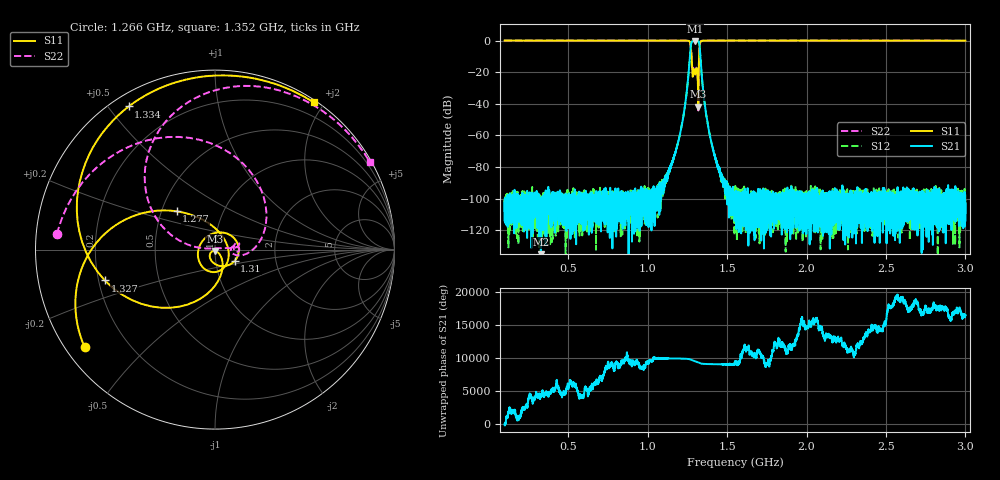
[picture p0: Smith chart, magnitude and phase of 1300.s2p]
# Hz S DB R 50
! Planar, S50180, 20087770, 20.1.2/1
! Date: 23.06.2021 14:42:37
! Data: Format (Calibration Info)
! Freq	S11:dB/Ang(F2)	S21:dB/Ang(F2)	S12:dB/Ang(F2)	S22:dB/Ang(F2)
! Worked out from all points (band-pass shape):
!   8991 points, 100 MHz to 3 GHz, reference 50 ohm
!   highest |S21| = -0.42 dB at 1.299 GHz (marker M1); lowest = -138.1 dB at 328.1 MHz (marker M2)
!   |S21| within 3 dB of the highest: 1.272 GHz to 1.327 GHz (55.52 MHz wide, 4.27 % of centre)
!   lowest |S11| = -41.8 dB at 1.319 GHz (marker M3), VSWR 1.02, Z = 49.9 - j0.794 ohm
!   |S11| at or under -10 dB: 1.277 GHz to 1.324 GHz (47.72 MHz wide, 3.67 % of centre)
!   |S22| runs from -44.2 to 0.0 dB; largest |S21 - S12| = 0.0016
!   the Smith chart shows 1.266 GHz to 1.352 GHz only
!   S11 on the Smith chart (normalised r, x): 1.266 GHz: 0.05, -0.33; 1.277 GHz: 0.60, +0.28; 1.31 GHz: 1.23, -0.16; 1.327 GHz: 0.23, -0.13; 1.334 GHz: 0.05, +0.56; 1.352 GHz: 0.03, +1.87
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1e8  0.02 154.0  -102.43 -44.0  -100.79 63.9  0.01 150.2
3.280645e8  -0.03 100.8  -138.06 -114.1  -105.57 -165.2  0.01 91.9
5.835484e8  -0.00 54.6  -99.35 47.0  -96.81 -103.7  0.01 45.4
1.066774e9  -0.00 -13.5  -98.83 -102.0  -100.61 -88.2  0.04 -18.9
1.138387e9  -0.00 -27.2  -80.94 -116.0  -81.34 -127.8  0.00 -32.0
1.172903e9  -0.02 -36.5  -71.66 -128.5  -71.10 -130.5  0.01 -41.0
1.242581e9  -0.07 -79.1  -35.65 -175.7  -35.64 -175.7  -0.07 -88.1
1.266129e9  -0.85 -143.2  -9.92 102.0  -9.92 102.0  -1.06 174.3
1.276774e9  -10.40 135.1  -1.03 -14.6  -1.04 -14.6  -10.41 22.7
1.28871e9  -18.49 -74.4  -0.46 -122.8  -0.47 -122.8  -18.00 7.8
1.299032e9  -21.49 131.0  -0.42 159.2  -0.42 159.1  -19.59 4.7
1.309677e9  -17.99 -30.3  -0.47 78.6  -0.47 78.5  -17.59 9.0
1.31871e9  -41.84 -100.1  -0.48 0.8  -0.49 0.8  -39.90 40.0
1.327419e9  -3.91 -164.3  -3.57 -105.3  -3.58 -105.3  -3.64 124.2
1.334194e9  -0.62 121.1  -13.25 -169.4  -13.26 -169.5  -0.49 73.1
1.351613e9  -0.11 56.1  -33.55 134.8  -33.55 134.8  -0.07 29.4
1.387419e9  -0.05 16.9  -57.76 100.4  -57.80 100.6  0.01 1.8
1.437742e9  -0.01 -4.2  -77.91 82.5  -78.59 83.2  0.01 -14.1
1.55e9  -0.01 -25.4  -99.99 75.4  -98.86 67.2  0.03 -32.1
2.033548e9  -0.04 -71.2  -94.16 -63.0  -104.25 -171.2  -0.01 -73.2
2.516774e9  -0.07 -107.4  -105.81 167.4  -102.80 158.4  -0.05 -106.3
3e9  -0.10 -143.3  -109.08 -80.7  -100.71 -140.5  -0.09 -139.7
